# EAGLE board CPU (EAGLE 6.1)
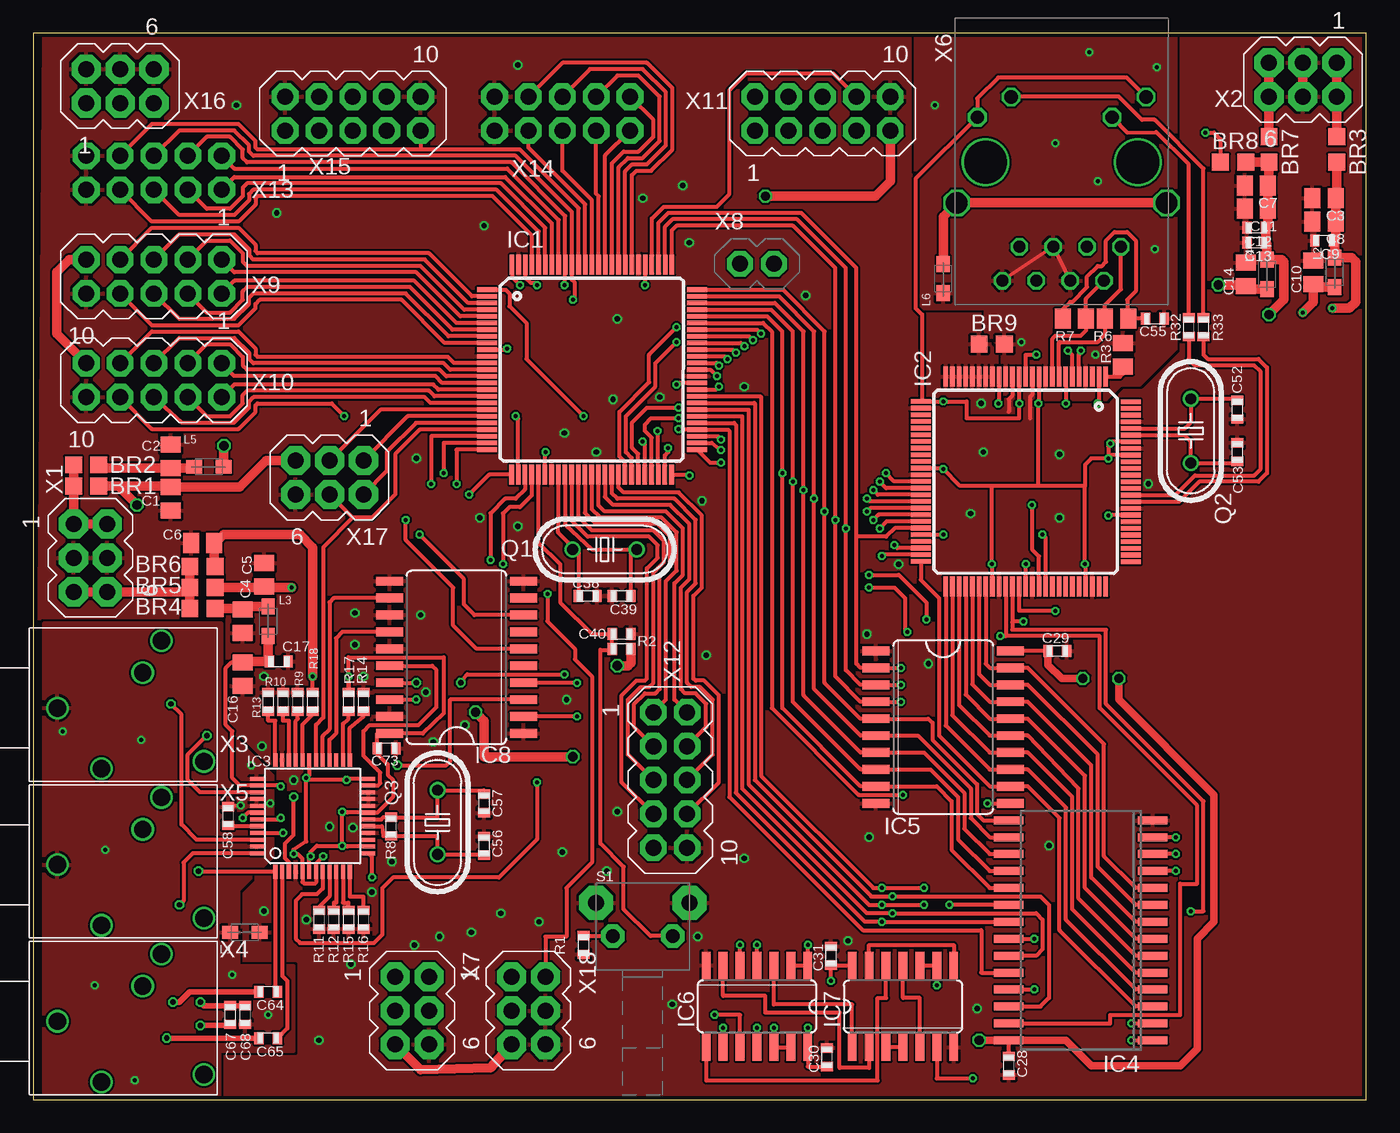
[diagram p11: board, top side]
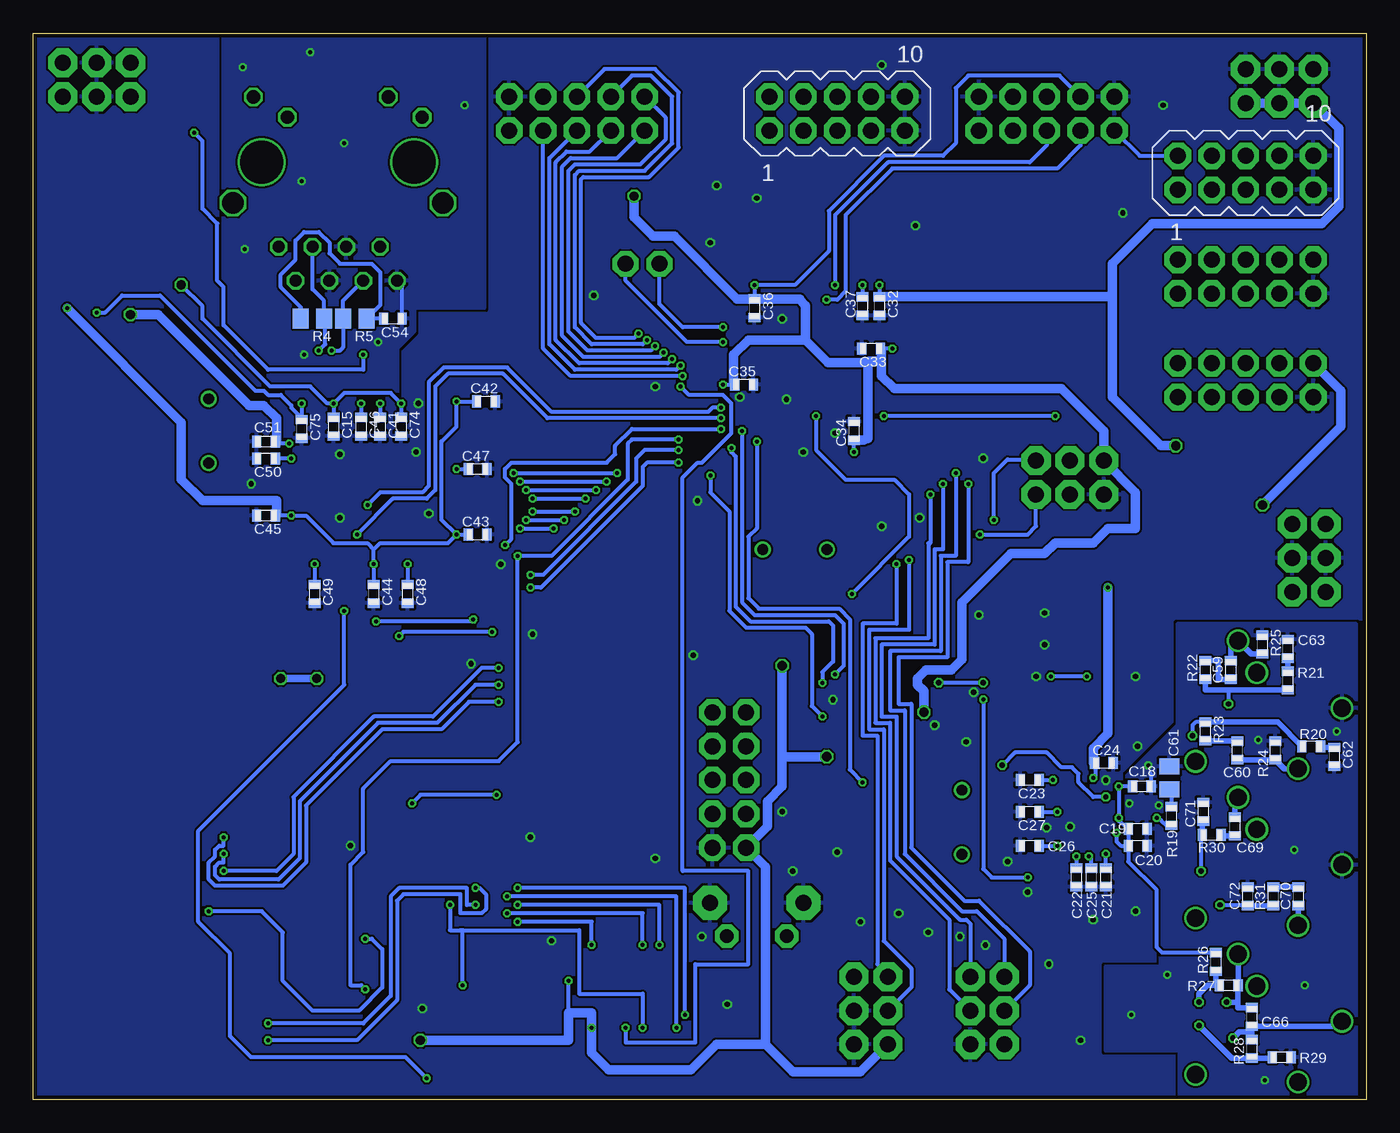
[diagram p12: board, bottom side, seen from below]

Size 100 x 80 mm. Coordinates in mm from the lower left corner, seen from the top.
Outline: 0,0 100,0 100,80 0,80 0,0
Copper layers (1*16): Top 0.035mm / dielectric 1.5mm / Bottom 0.035mm
Design rules: minimum track width 0.15mm, minimum drill 0.3mm, track to track 0.15mm, track to pad 0.15mm, pad to pad 0.15mm, via to via 0.15mm, smd to smd 0.15mm, copper to edge 0.3mm, drill to drill 0.2mm, minimum pad ring 0.2mm, minimum via ring 0.15mm, stop-mask expansion 0.075mm, vias tented up to drill 0mil, thermal gap 0.2mm

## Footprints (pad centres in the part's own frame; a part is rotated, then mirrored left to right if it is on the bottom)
0-OHM-BRÜCKE = smd 1.27 x 1.27: 1 -0.953,0; 2 0.953,0
0805 = smd 1.2 x 1.5: 1 -0.875,0; 2 0.875,0
0603 = smd 0.7 x 0.9: 1 -0.7,0; 2 0.7,0
TQFP100 = smd 1.5 x 0.35: 1 -7.875,6; 2 -7.875,5.5; 3 -7.875,5; 4 -7.875,4.5; 5 -7.875,4; 6 -7.875,3.5; 7 -7.875,3; 8 -7.875,2.5; 9 -7.875,2; 10 -7.875,1.5; 11 -7.875,1; 12 -7.875,0.5; 13 -7.875,0; 14 -7.875,-0.5; 15 -7.875,-1; 16 -7.875,-1.5; 17 -7.875,-2; 18 -7.875,-2.5; 19 -7.875,-3; 20 -7.875,-3.5; 21 -7.875,-4; 22 -7.875,-4.5; 23 -7.875,-5; 24 -7.875,-5.5; 25 -7.875,-6; 51 7.875,-6; 52 7.875,-5.5; 53 7.875,-5; 54 7.875,-4.5; 55 7.875,-4; 56 7.875,-3.5; 57 7.875,-3; 58 7.875,-2.5; 59 7.875,-2; 60 7.875,-1.5; 61 7.875,-1; 62 7.875,-0.5; 63 7.875,0; 64 7.875,0.5; 65 7.875,1; 66 7.875,1.5; 67 7.875,2; 68 7.875,2.5; 69 7.875,3; 70 7.875,3.5; 71 7.875,4; 72 7.875,4.5; 73 7.875,5; 74 7.875,5.5; 75 7.875,6 | smd 0.35 x 1.5: 26 -6.025,-7.875; 27 -5.525,-7.875; 28 -5.025,-7.875; 29 -4.525,-7.875; 30 -4.025,-7.875; 31 -3.525,-7.875; 32 -3.025,-7.875; 33 -2.525,-7.875; 34 -2.025,-7.875; 35 -1.525,-7.875; 36 -1.025,-7.875; 37 -0.525,-7.875; 38 -0.025,-7.875; 39 0.475,-7.875; 40 0.975,-7.875; 41 1.475,-7.875; 42 1.975,-7.875; 43 2.475,-7.875; 44 2.975,-7.875; 45 3.475,-7.875; 46 3.975,-7.875; 47 4.475,-7.875; 48 4.975,-7.875; 49 5.475,-7.875; 50 5.975,-7.875; 76 6,7.875; 77 5.5,7.875; 78 5,7.875; 79 4.5,7.875; 80 4,7.875; 81 3.5,7.875; 82 3,7.875; 83 2.5,7.875; 84 2,7.875; 85 1.5,7.875; 86 1,7.875; 87 0.5,7.875; 88 0,7.875; 89 -0.5,7.875; 90 -1,7.875; 91 -1.5,7.875; 92 -2,7.875; 93 -2.5,7.875; 94 -3,7.875; 95 -3.5,7.875; 96 -4,7.875; 97 -4.5,7.875; 98 -5,7.875; 99 -5.5,7.875; 100 -6,7.875
TQFP48 = smd 1.016 x 0.305: 1 -4.191,2.794; 2 -4.191,2.286; 3 -4.191,1.778; 4 -4.191,1.27; 5 -4.191,0.762; 6 -4.191,0.254; 7 -4.191,-0.254; 8 -4.191,-0.762; 9 -4.191,-1.27; 10 -4.191,-1.778; 11 -4.191,-2.286; 12 -4.191,-2.794; 25 4.191,-2.794; 26 4.191,-2.286; 27 4.191,-1.778; 28 4.191,-1.27; 29 4.191,-0.762; 30 4.191,-0.254; 31 4.191,0.254; 32 4.191,0.762; 33 4.191,1.27; 34 4.191,1.778; 35 4.191,2.286; 36 4.191,2.794 | smd 0.305 x 1.016: 13 -2.794,-4.191; 14 -2.286,-4.191; 15 -1.778,-4.191; 16 -1.27,-4.191; 17 -0.762,-4.191; 18 -0.254,-4.191; 19 0.254,-4.191; 20 0.762,-4.191; 21 1.27,-4.191; 22 1.778,-4.191; 23 2.286,-4.191; 24 2.794,-4.191; 37 2.794,4.191; 38 2.286,4.191; 39 1.778,4.191; 40 1.27,4.191; 41 0.762,4.191; 42 0.254,4.191; 43 -0.254,4.191; 44 -0.762,4.191; 45 -1.27,4.191; 46 -1.778,4.191; 47 -2.286,4.191; 48 -2.794,4.191
SOP28X = smd 0.6 x 2.2: 1 -8.255,-5.4; 2 -6.985,-5.4; 3 -5.715,-5.4; 4 -4.445,-5.4; 5 -3.175,-5.4; 6 -1.905,-5.4; 7 -0.635,-5.4; 8 0.635,-5.4; 9 1.905,-5.4; 10 3.175,-5.4; 11 4.445,-5.4; 12 5.715,-5.4; 13 6.985,-5.4; 14 8.255,-5.4; 15 8.255,5.4; 16 6.985,5.4; 17 5.715,5.4; 18 4.445,5.4; 19 3.175,5.4; 20 1.905,5.4; 21 0.635,5.4; 22 -0.635,5.4; 23 -1.905,5.4; 24 -3.175,5.4; 25 -4.445,5.4; 26 -5.715,5.4; 27 -6.985,5.4; 28 -8.255,5.4
SO20W = smd 0.66 x 2.032: 1 -5.715,-5.029; 2 -4.445,-5.029; 3 -3.175,-5.029; 4 -1.905,-5.029; 5 -0.635,-5.029; 6 0.635,-5.029; 7 1.905,-5.029; 8 3.175,-5.029; 9 4.445,-5.029; 10 5.715,-5.029; 11 5.715,5.029; 12 4.445,5.029; 13 3.175,5.029; 14 1.905,5.029; 15 0.635,5.029; 16 -0.635,5.029; 17 -1.905,5.029; 18 -3.175,5.029; 19 -4.445,5.029; 20 -5.715,5.029
SO14 = smd 0.66 x 2.032: 1 -3.81,-3.073; 2 -2.54,-3.073; 3 -1.27,-3.073; 4 0,-3.073; 5 1.27,-3.073; 6 2.54,-3.073; 7 3.81,-3.073; 8 3.81,3.073; 9 2.54,3.073; 10 1.27,3.073; 11 0,3.073; 12 -1.27,3.073; 13 -2.54,3.073; 14 -3.81,3.073
0805' = smd 1.2 x 1: 1 -1.1,0; 2 1.1,0
HC49U-V = drill 0.813: 1 -2.413,0; 2 2.413,0
PHAP3305 = drill 1 pad 1.778 octagon: 1 -2.25,-2.5; 2 2.25,-2.5 | drill 1.2 pad 2.54 octagon: SHD@0 -3.5,0; SHD@1 3.5,0
STIFTLEISTE-2X3PIN = drill 1.2 pad 2.184 octagon: 1 -2.54,-2.54; 2 0,-2.54; 3 2.54,-2.54; 4 -2.54,0; 5 0,0; 6 2.54,0
EBS35 = drill 1.3: GND -12,0; LEFT -4.2,5.05; LEFTGND -5.6,2.65; RIGHT -8.7,-4.55; RIGHTGND -1,-4
TRJ0011 = drill 0.9 octagon: 1 4.445,-6.35; 2 3.175,-8.89; 3 1.905,-6.35; 4 0.635,-8.89; 5 -0.635,-6.35; 6 -1.905,-8.89; 7 -3.175,-6.35; 8 -4.445,-8.89 | drill 1 octagon: 9 6.325,4.9; 10 3.785,3.38; 11 -3.785,4.9; 12 -6.325,3.38 | drill 3.2 pad 3.2: P$1 -5.715,0; P$2 5.715,0 | drill 1.6 octagon: SHD@0 -7.875,-3.05; SHD@1 7.875,-3.05
STIFTLEISTE-2PIN = drill 1.2 pad 1.93 octagon: 1 0,0; 2 2.54,0
STIFTLEISTE-2X5PIN = drill 1.2 pad 2 octagon: 1 -5.08,-2.54; 2 -2.54,-2.54; 3 0,-2.54; 4 2.54,-2.54; 5 5.08,-2.54; 6 -5.08,0; 7 -2.54,0; 8 0,0; 9 2.54,0; 10 5.08,0

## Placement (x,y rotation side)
BR1  0-OHM-BRÜCKE  [0-OHM-BRÜCKE]  3.97,46.04 0 top
BR2  0-OHM-BRÜCKE  [0-OHM-BRÜCKE]  3.97,47.62 0 top
BR3  0-OHM-BRÜCKE  [0-OHM-BRÜCKE]  97.79,71.28 270 top
BR4  0-OHM-BRÜCKE  [0-OHM-BRÜCKE]  12.7,36.83 0 top
BR5  0-OHM-BRÜCKE  [0-OHM-BRÜCKE]  12.7,38.42 0 top
BR6  0-OHM-BRÜCKE  [0-OHM-BRÜCKE]  12.7,40.01 0 top
BR7  0-OHM-BRÜCKE  [0-OHM-BRÜCKE]  92.71,71.28 270 top
BR8  0-OHM-BRÜCKE  [0-OHM-BRÜCKE]  90.01,70.33 0 top
BR9  0-OHM-BRÜCKE  [0-OHM-BRÜCKE]  71.91,56.67 0 top
C1  10µF  [0805]  10.32,45.09 270 top
C2  10µF  [0805]  10.32,48.26 90 top
C3  10µF  [0805]  96.84,67.63 180 top
C4  10µF  [0805]  15.72,35.88 270 top
C5  10µF  [0805]  17.3,39.37 90 top
C6  10µF  [0805]  12.7,41.75 180 top
C7  10µF  [0805]  91.76,68.58 180 top
C8  10µF  [0805]  96.84,65.88 180 top
C9  0µ1F  [0603]  96.84,64.45 180 top
C10  10µF  [0805]  96.04,62.07 90 top
C11  10µF  [0805]  91.76,66.83 180 top
C12  3µ3F  [0603]  91.76,65.41 180 top
C13  0µ1F  [0603]  91.76,64.29 180 top
C14  10µF  [0805]  90.96,61.91 90 top
C15  0µ1F  [0603]  77.47,50.48 270 bottom
C16  10µF  [0805]  15.72,31.91 270 top
C17  0µ1F  [0603]  18.41,32.86 0 top
C18  0µ1F  [0603]  16.83,23.5 0 bottom
C19  0µ1F  [0603]  17.14,20.32 0 bottom
C20  0µ1F  [0603]  17.14,19.05 0 bottom
C21  0µ1F  [0603]  19.53,16.67 270 bottom
C22  0µ1F  [0603]  21.75,16.67 270 bottom
C23  0µ1F  [0603]  25.24,23.97 180 bottom
C24  0µ1F  [0603]  19.68,25.24 0 bottom
C25  0µ1F  [0603]  20.64,16.67 270 bottom
C26  0µ1F  [0603]  25.24,19.05 180 bottom
C27  0µ1F  [0603]  25.24,21.59 180 bottom
C28  0µ1F  [0603]  73.18,2.54 270 top
C29  0µ1F  [0603]  76.83,33.66 0 top
C30  0µ1F  [0603]  59.53,3.17 90 top
C31  0µ1F  [0603]  59.85,10.79 90 top
C32  0µ1F  [0603]  36.51,59.53 270 bottom
C33  0µ1F  [0603]  37.15,56.36 180 bottom
C34  0µ1F  [0603]  38.42,50.16 90 bottom
C35  0µ1F  [0603]  46.67,53.66 0 bottom
C36  0µ1F  [0603]  45.88,59.37 270 bottom
C37  0µ1F  [0603]  37.78,59.53 270 bottom
C38  22pF  [0603]  41.59,37.78 0 top
C39  22pF  [0603]  44.13,37.78 180 top
C40  0µ1F  [0603]  44.13,34.92 0 top
C41  0µ1F  [0603]  73.98,50.48 270 bottom
C42  0µ1F  [0603]  66.04,52.39 0 bottom
C43  0µ1F  [0603]  66.67,42.39 0 bottom
C44  0µ1F  [0603]  74.45,37.94 270 bottom
C45  0µ1F  [0603]  82.55,43.81 180 bottom
C46  0µ1F  [0603]  75.41,50.48 270 bottom
C47  0µ1F  [0603]  66.67,47.31 0 bottom
C48  0µ1F  [0603]  71.91,37.94 270 bottom
C49  0µ1F  [0603]  78.9,37.94 270 bottom
C50  0µ1F  [0603]  82.55,48.1 180 bottom
C51  0µ1F  [0603]  82.55,49.37 180 bottom
C52  22pF  [0603]  90.33,51.75 90 top
C53  22pF  [0603]  90.33,48.58 270 top
C54  0µ1F  [0603]  73.03,58.58 180 bottom
C55  0µ1F  [0603]  84.14,58.58 0 top
C56  33pF  [0603]  33.81,19.05 90 top
C57  33pF  [0603]  33.81,22.23 270 top
C58  1µF  [0603]  14.61,21.27 90 top
C59  1µF  [0603]  10.16,32.23 90 bottom
C60  1µF  [0603]  9.68,26.19 270 bottom
C61  47nF  [0805]  14.76,24.13 90 bottom
C62  10nF  [0603]  2.38,25.72 270 bottom
C63  10nF  [0603]  5.87,33.81 90 bottom
C64  1µF  [0603]  17.62,8.1 180 top
C65  1µF  [0603]  17.62,4.6 180 top
C66  100pF  [0603]  8.57,6.19 270 bottom
C67  10µF  [0603]  14.76,6.35 270 top
C68  10µF  [0603]  15.88,6.35 270 top
C69  1µF  [0603]  9.84,20.48 90 bottom
C70  1µF  [0603]  5.08,15.24 270 bottom
C71  10nF  [0603]  12.22,21.59 90 bottom
C72  10nF  [0603]  8.89,15.24 90 bottom
C73  0µ1F  [0603]  26.51,26.35 0 top
C74  0µ1F  [0603]  72.39,50.48 270 bottom
C75  0µ1F  [0603]  79.85,50.32 270 bottom
IC1  ATMEGA-2560  [TQFP100]  41.91,54.77 0 top
IC2  W5300  [TQFP100]  74.45,46.35 270 top
IC3  VS1053B  [TQFP48]  20.95,21.27 90 top
IC4  62256-70M  [SOP28X]  78.58,12.7 90 top
IC5  74VHC573D  [SO20W]  68.26,27.94 270 top
IC6  7400  [SO14]  54.29,6.99 180 top
IC7  7400  [SO14]  65.25,6.99 0 top
IC8  74HCT244DW  [SO20W]  31.75,33.18 90 top
L1  1µH  [0805']  15.88,12.54 0 top
L2  1µH  [0805']  97.63,62.07 270 top
L3  1µH  [0805']  17.62,35.88 270 top
L4  1µH  [0805']  92.55,61.91 270 top
L5  10µH  [0805']  13.18,47.47 0 top
L6  120R Ferrit  [0805']  68.26,61.59 90 top
Q1  16 MHz  [HC49U-V]  42.86,41.27 0 top
Q2  25MHz  [HC49U-V]  86.84,50.16 270 top
Q3  12.288  [HC49U-V]  30.32,20.8 90 top
R1  100R  [0603]  41.27,11.59 90 top
R2  10K  [0603]  44.13,33.81 180 top
R3  12K3  [0805]  81.76,55.88 90 top
R4  49R9  [0805]  79.06,58.58 180 bottom
R5  49R9  [0805]  75.88,58.58 0 bottom
R6  49R9  [0805]  81.28,58.58 180 top
R7  49R9  [0805]  78.11,58.58 0 top
R8  1M  [0603]  26.83,20.48 90 top
R9  100K  [0603]  19.84,29.84 270 top
R10  100K  [0603]  18.73,29.84 270 top
R11  100K  [0603]  21.43,13.49 90 top
R12  100K  [0603]  22.54,13.49 90 top
R13  100K  [0603]  17.62,29.84 270 top
R14  100K  [0603]  24.77,29.84 270 top
R15  100K  [0603]  23.65,13.49 90 top
R16  100K  [0603]  24.77,13.49 90 top
R17  100K  [0603]  23.65,29.84 270 top
R18  100K  [0603]  20.95,29.84 270 top
R19  10R  [0603]  14.61,21.27 270 bottom
R20  22R  [0603]  4.13,26.51 180 bottom
R21  22R  [0603]  5.87,31.43 270 bottom
R22  100R  [0603]  12.06,32.23 90 bottom
R23  100R  [0603]  12.06,27.62 270 bottom
R24  10K  [0603]  6.83,26.19 270 bottom
R25  10K  [0603]  7.78,34.13 270 bottom
R26  1K  [0603]  11.27,10.32 90 bottom
R27  1K  [0603]  10.32,8.57 180 bottom
R28  1K  [0603]  8.57,3.81 90 bottom
R29  1K  [0603]  6.35,3.17 180 bottom
R30  470R  [0603]  11.59,19.84 0 bottom
R31  470R  [0603]  6.99,15.24 90 bottom
R32  220R  [0603]  86.68,57.94 90 top
R33  220R  [0603]  87.79,57.94 90 top
S1  PHAP3305  [PHAP3305]  45.72,14.76 0 top
X1  VIN  [STIFTLEISTE-2X3PIN]  5.56,40.64 270 top
X2  VIN  [STIFTLEISTE-2X3PIN]  95.25,75.25 180 top
X3  DS_1503_09  [EBS35]  13.81,29.37 0 top
X4  DS_1503_09  [EBS35]  13.81,5.87 0 top
X5  DS_1503_09  [EBS35]  13.81,17.62 0 top
X6  TRJ0011  [TRJ0011]  77.15,70.33 0 top
X7  PB  [STIFTLEISTE-2X3PIN]  29.69,6.67 270 top
X8  TWI  [STIFTLEISTE-2PIN]  53.02,62.71 0 top
X9  PE  [STIFTLEISTE-2X5PIN]  9.05,60.48 180 top
X10  PH  [STIFTLEISTE-2X5PIN]  9.05,52.7 180 top
X11  PJ  [STIFTLEISTE-2X5PIN]  59.21,75.25 0 top
X12  PL  [STIFTLEISTE-2X5PIN]  49.05,23.97 270 top
X13  PF  [STIFTLEISTE-2X5PIN]  9.05,70.8 0 bottom
X14  PK  [STIFTLEISTE-2X5PIN]  39.69,75.25 0 bottom
X15  JTAG  [STIFTLEISTE-2X5PIN]  23.97,75.25 0 top
X16  ADC Supply  [STIFTLEISTE-2X3PIN]  6.51,77.31 0 top
X17  SPI  [STIFTLEISTE-2X3PIN]  22.23,45.4 180 top
X18  PG  [STIFTLEISTE-2X3PIN]  38.42,6.67 270 top

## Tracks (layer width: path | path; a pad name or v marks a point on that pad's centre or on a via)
1V8O  (via drill 0.3)
  Top 0.3: IC2.13 74.45,55.88 v75.25,55.88 | v87.95,72.55 88.58,72.55 89.06,72.07 BR8.1
  Bottom 0.3: v75.25,55.88 75.25,54.77 82.39,54.77 85.72,58.1 85.72,60.96 86.2,61.44 86.2,65.72 87.31,66.83 87.31,71.91 v87.95,72.55
3V3
  Top 0.7: X2.1 X2.4 BR3.1
!FDX
  Top 0.3: IC2.86 85.68,45.35 87.15,46.83 91.6,46.83 92.08,47.31 92.08,54.61 91.6,55.09 87.15,55.09 86.68,55.56 R32.1
!RD  (via drill 0.3)
  Top 0.3: IC1.52 50.9,49.27 v51.59,48.74 | IC4.22 v75.09,12.06 | v86.84,14.13 87.79,14.13 87.79,22.38 80.49,29.69 80.49,35.24 73.45,35.24 73.45,35.83 | IC2.61 73.45,35.83 | v62.71,39.37 64.93,39.37 66.99,37.31 v66.99,36.04 | v74.3,35.88 73.5,35.88 73.45,35.83
  Bottom 0.3: v51.59,48.74 54.13,48.74 54.77,48.1 54.77,46.35 61.75,39.37 v62.71,39.37 | v75.09,12.06 74.61,12.06 73.82,11.27 73.82,8.41 75.56,6.67 79.06,6.67 81.28,8.89 81.28,12.54 82.87,14.13 v86.84,14.13 | v66.99,36.04 67.15,35.88 v74.3,35.88
!SPD
  Top 0.3: R33.1 87.79,55.88 88.11,55.56 91.92,55.56 92.55,54.93 92.55,46.99 91.92,46.35 87.47,46.35 85.97,44.85 IC2.85
!WR  (via drill 0.3)
  Top 0.3: IC4.27 80.8,5.71 80.8,6.35 86.04,6.35 86.04,16.19 87.31,16.19 87.31,22.07 80.01,29.37 80.01,34.77 72.95,34.77 | IC2.60 72.95,34.77 | IC1.51 50.77,47.78 v51.59,47.78 | v62.71,38.42 64.61,38.42 65.41,37.62 65.41,35.24 v65.56,35.08 | v72.55,34.77 72.95,34.77
  Bottom 0.3: v51.59,47.78 53.98,47.78 54.29,47.47 54.29,46.04 61.91,38.42 v62.71,38.42 | v65.56,35.08 72.23,35.08 v72.55,34.77
+1V8
  Top 0.7: X2.3 X2.6 BR7.1
+3V3
  Top 0.7: X1.3 X1.6 11.43,38.1 BR5.1 | BR5.1 BR4.1 | BR5.1 BR6.1
+5V
  Top 0.7: BR2.1 BR1.1 X1.1 X1.4
A0
  Top 0.3: IC2.57 71.45,32.69 71.75,32.38 IC5.19 74.61,32.38 80.33,26.67 80.33,18.26 82.71,15.88 IC4.10
A1
  Top 0.3: IC2.56 70.95,31.92 71.75,31.11 IC5.18 74.61,31.11 79.85,25.88 79.85,17.46 82.71,14.61 IC4.9
A2
  Top 0.3: IC2.55 70.45,31.15 71.75,29.84 IC5.17 74.61,29.84 79.38,25.08 79.38,16.67 82.71,13.34 IC4.8
A3
  Top 0.3: IC2.54 69.95,30.38 71.75,28.57 IC5.16 74.61,28.57 78.9,24.29 78.9,15.88 82.71,12.06 IC4.7
A4
  Top 0.3: IC2.53 69.45,29.61 71.75,27.3 IC5.15 74.61,27.3 78.42,23.34 78.42,15.08 82.71,10.79 IC4.6
A5
  Top 0.3: IC2.52 68.95,28.84 71.75,26.04 IC5.14 74.61,26.04 77.95,22.7 77.95,14.29 82.71,9.53 IC4.5
A6
  Top 0.3: IC2.51 68.45,28.07 71.75,24.77 IC5.13 74.61,24.77 77.47,21.91 77.47,13.49 82.71,8.26 IC4.4
A7
  Top 0.3: IC2.50 66.58,38.99 67.94,37.62 67.94,27.3 71.75,23.5 IC5.12 74.61,23.5 76.99,21.11 76.99,12.7 82.71,6.99 IC4.3
A8  (via drill 0.3)
  Top 0.3: IC2.49 63.74,40.88 v63.66,40.8 | IC1.53 51.35,49.77 v51.59,49.53 | IC4.25 v75.09,8.26
  Bottom 0.3: v51.59,49.53 55.09,49.53 55.4,49.21 55.4,46.51 61.12,40.8 v63.66,40.8 63.66,26.83 65.09,25.4 73.18,25.4 75.25,23.34 75.25,18.57 76.2,17.62 76.2,8.57 75.41,8.57 v75.09,8.26
A9  (via drill 0.3)
  Top 0.3: IC4.24 71.12,9.53 71.12,12.7 62.23,12.7 52.23,22.7 52.23,50.16 52.12,50.27 IC1.54 48.47,50.27 v48.42,50.32 | IC2.48 64.82,41.38 v64.61,41.59
  Bottom 0.3: v64.61,41.59 64.14,42.07 64.14,46.2 64.61,46.67 64.61,47.31 64.14,47.78 56.99,47.78 56.36,48.42 56.36,49.05 55.09,50.32 v48.42,50.32
A10  (via drill 0.3)
  Top 0.3: IC1.55 52.58,50.77 52.7,50.64 52.7,23.02 62.39,13.34 v63.66,13.34 IC4.21 | IC6.2 IC6.1 v58.1,11.59
  Bottom 0.3: v58.1,11.59 58.1,13.34 v63.66,13.34
A11  (via drill 0.3)
  Top 0.3: IC1.56 53.17,51.27 53.18,51.28 53.18,23.34 62.55,13.97 v64.45,13.97 75.25,13.97 75.72,13.49 75.72,11.27 75.25,10.79 IC4.23 | IC6.4 v54.29,11.59
  Bottom 0.3: v54.29,11.59 54.29,13.97 v64.45,13.97
A12  (via drill 0.3)
  Top 0.3: IC1.57 53.64,51.77 53.66,51.75 53.66,23.65 62.71,14.61 v63.66,14.61 v66.83,14.61 | v82.39,5.71 IC4.2 | IC6.5 v53.02,11.59
  Bottom 0.3: v66.83,14.61 67.47,14.61 67.47,15.88 72.55,15.88 73.18,15.24 73.18,7.78 75.25,5.71 v82.39,5.71 | v53.02,11.59 53.02,14.61 v63.66,14.61
A13  (via drill 0.3)
  Top 0.3: IC1.58 54.09,52.27 54.13,52.23 54.13,23.97 62.87,15.24 v64.45,15.24 75.56,15.24 76.2,14.61 76.2,7.62 75.56,6.99 IC4.26 | IC6.9 v51.75,5.4
  Bottom 0.3: v51.75,5.4 51.75,15.24 v64.45,15.24
A14  (via drill 0.3)
  Top 0.3: IC1.59 54.55,52.77 54.61,52.7 54.61,24.29 63.02,15.88 v63.66,15.88 v66.83,15.88 | v82.39,4.45 IC4.1 | IC6.10 53.02,6.35 v51.12,6.35
  Bottom 0.3: v66.83,15.88 66.52,15.88 66.04,15.4 66.04,14.29 66.36,13.97 67.94,13.97 67.94,15.4 72.23,15.4 72.71,14.92 72.71,7.46 75.72,4.45 v82.39,4.45 | v51.12,6.35 51.12,15.88 v63.66,15.88
A15  (via drill 0.3)
  Top 0.3: IC6.13 IC6.12 v55.56,5.4 | 51.28,53.34 v51.44,53.5 51.2,53.27 IC1.60
  Bottom 0.3: v55.56,5.4 55.56,4.29 50.32,4.29 50.32,10.16 46.35,10.16 46.35,17.14 51.28,17.14 51.28,46.67 50.16,47.78 49.85,47.78 47.62,50.01 47.62,52.23 48.26,52.86 50.8,52.86 v51.44,53.5
AD0  (via drill 0.3)
  Top 0.3: 61.75,42.23 61.75,32.7 62.07,32.38 IC5.2 v65.09,32.38 | 61.75,42.23 61.75,62.39 57.63,66.52 47.62,66.52 46.91,65.8 IC1.78 | IC2.45 64.63,42.88 63.98,42.23 61.75,42.23 | v85.72,17.14 IC4.11
  Bottom 0.3: v65.09,32.38 66.36,32.38 70.01,28.73 74.45,28.73 80.49,22.7 80.49,18.41 81.76,17.14 v85.72,17.14
AD1  (via drill 0.3)
  Top 0.3: IC1.77 47.41,65.51 47.94,66.04 57.31,66.04 60.96,62.39 v60.96,42.86 60.96,32.23 62.07,31.11 IC5.3 v65.09,31.11 | IC2.44 64.02,43.38 v63.5,42.86 | v85.72,18.41 IC4.12
  Bottom 0.3: v63.5,42.86 v60.96,42.86 | v65.09,31.11 66.83,31.11 69.69,28.26 74.14,28.26 80.01,22.38 80.01,18.1 81.6,16.51 86.04,16.51 86.36,16.83 86.36,17.46 86.04,17.78 85.72,17.78 v85.72,18.41
AD2  (via drill 0.3)
  Top 0.3: IC1.76 47.91,65.21 48.26,65.56 56.99,65.56 60.17,62.39 v60.17,43.5 60.17,31.75 62.07,29.84 IC5.4 v65.09,29.84 | IC2.43 63.41,43.88 v63.02,43.5 | v85.72,19.68 IC4.13
  Bottom 0.3: v63.02,43.5 v60.17,43.5 | v65.09,29.84 67.31,29.84 69.37,27.78 73.82,27.78 79.53,22.07 79.53,17.78 81.28,16.03 86.36,16.03 86.84,16.51 86.84,17.78 86.36,18.26 86.36,18.73 86.04,19.05 85.72,19.05 v85.72,19.68
AD3  (via drill 0.3)
  Top 0.3: IC1.75 56.23,60.77 59.37,57.63 v59.37,44.13 59.37,31.27 62.07,28.57 IC5.5 67.15,28.57 67.47,28.26 67.47,26.99 70.8,23.65 70.8,21.43 71.28,20.95 IC4.15 | IC2.42 62.8,44.38 v62.55,44.13
  Bottom 0.3: v62.55,44.13 v59.37,44.13
AD4  (via drill 0.3)
  Top 0.3: IC1.74 55.94,60.27 58.58,57.63 v58.58,45.09 58.58,30.8 62.07,27.3 IC5.6 66.36,27.3 70.33,23.34 70.33,21.11 71.75,19.68 IC4.16 | IC2.41 62.75,44.88 v62.55,45.09
  Bottom 0.3: v62.55,45.09 v58.58,45.09
AD5  (via drill 0.3)
  Top 0.3: IC1.73 55.64,59.77 57.78,57.63 v57.78,45.72 57.78,30.32 62.07,26.04 IC5.7 66.83,26.04 69.85,23.02 69.85,20.32 71.75,18.41 IC4.17 | IC2.40 63.36,45.38 v63.02,45.72
  Bottom 0.3: v63.02,45.72 v57.78,45.72
AD6  (via drill 0.3)
  Top 0.3: IC1.72 55.35,59.27 56.99,57.63 v56.99,46.35 56.99,29.84 62,24.84 arc45 62.18,24.77 IC5.8 67.31,24.77 69.37,22.7 69.37,19.53 71.75,17.14 IC4.18 | IC2.39 63.98,45.88 v63.5,46.35
  Bottom 0.3: v63.5,46.35 v56.99,46.35
AD7  (via drill 0.3)
  Top 0.3: IC1.71 55.05,58.77 56.2,57.63 v56.2,46.99 56.2,29.37 62.07,23.5 IC5.9 67.79,23.5 68.9,22.38 68.9,18.73 71.75,15.88 IC4.19 | IC2.38 64.59,46.38 v63.98,46.99
  Bottom 0.3: v63.98,46.99 v56.2,46.99
ADC0
  Top 0.3: IC1.97 37.41,64.83 34.45,67.79 16.83,67.79 16.67,67.63 16.67,67.15 15.4,65.88 8.89,65.88 X13.4
ADC1
  Top 0.3: IC1.96 37.91,65.12 34.77,68.26 16.51,68.26 16.19,67.94 16.19,67.47 15.08,66.36 10.95,66.36 X13.3
ADC2
  Top 0.3: IC1.95 38.41,65.41 35.08,68.74 16.03,68.74 15.72,68.42 15.72,67.79 14.76,66.83 13.02,66.83 X13.2
ADC3
  Top 0.3: X13.1 15.08,69.22 35.4,69.22 38.91,65.71 IC1.94
ADC4
  Top 0.3: X13.6 15.08,69.85 35.56,69.85 39.41,66 IC1.93
  Bottom 0.3: X15.1 16.99,70.8 X13.6
ADC5  (via drill 0.3)
  Top 0.3: X13.7 13.02,72.23 14.76,72.23 15.72,71.28 15.72,70.64 16.03,70.33 35.88,70.33 39.91,66.29 IC1.92 39.91,61.18 v39.85,61.12
  Bottom 0.3: X15.3 23.97,71.6 25.24,70.33 35.88,70.33 39.85,66.36 v39.85,61.12
ADC6  (via drill 0.3)
  Top 0.3: X13.8 10.95,72.71 15.08,72.71 16.19,71.6 16.19,71.12 16.51,70.8 36.2,70.8 40.41,66.59 IC1.91 40.41,61.51 40.64,61.28 40.64,60.17 v40.48,60.01
  Bottom 0.3: X15.2 21.43,71.6 23.18,69.85 35.56,69.85 39.05,66.36 39.05,60.64 39.69,60.01 v40.48,60.01
ADC7
  Top 0.3: IC1.90 40.91,66.88 36.51,71.28 29.05,71.28 | 29.05,71.28 16.83,71.28 16.67,71.44 16.67,71.91 15.4,73.18 8.89,73.18 X13.9 | X15.5 29.05,71.28
ADC8
  Top 0.3: IC1.89 41.41,67.17 37.15,71.44 X14.4
ADC9
  Top 0.3: IC1.88 41.91,67.47 39.69,69.69 X14.3
ADC10
  Top 0.3: IC1.87 42.41,67.76 42.23,67.94 X14.2
ADC11
  Top 0.3: IC1.86 42.91,70.85 X14.1
ADC12
  Top 0.3: IC1.85 43.41,70.24 44.29,71.12 45.4,71.12 46.51,72.23 46.51,73.5 X14.6
ADC13
  Top 0.3: IC1.84 43.91,69.94 44.61,70.64 45.72,70.64 46.99,71.91 46.99,75.25 45.4,76.83 43.81,76.83 X14.7
ADC14
  Top 0.3: IC1.83 44.41,69.65 44.93,70.17 46.04,70.17 47.47,71.6 47.47,75.56 45.72,77.31 41.75,77.31 X14.8
ADC15
  Top 0.3: IC1.82 44.91,69.36 45.24,69.69 46.35,69.69 47.94,71.28 47.94,75.88 46.04,77.79 39.69,77.79 X14.9
AGND  (via drill 0.3)
  Top 0.3: C58.2 14.86,22.07 v15.56,22.07
  Bottom 0.3: C18.2 16.13,24.38 16.19,24.45
  other vias: 14.92,9.37 17.62,6.35 7.62,1.43 4.6,8.57 5.4,18.73 8.1,26.99 2.22,27.62 17.78,22.23 16.35,25.08
  pour Bottom: 0.79,0.16 13.97,0.16 13.97,3.65 19.53,3.65 19.53,10 15.4,10 15.4,15.72 17.94,18.26 17.94,24.29 14.13,28.1 14.13,35.72 0.79,35.72
  pour Top: 0.79,0.16 13.97,0.16 13.97,3.65 19.53,3.65 19.53,10 15.4,10 15.4,15.72 17.94,18.26 17.94,24.29 14.13,28.1 14.13,35.72 0.79,35.72
ALE  (via drill 0.3)
  Top 0.3: IC1.70 54.76,58.27 55.4,57.63 55.4,29.37 61.91,22.86 v65.25,22.86 | v71.6,22.23 IC5.11
  Bottom 0.3: v65.25,22.86 70.96,22.86 v71.6,22.23
AVCC  (via drill 0.3, 0.7)
  Top 0.3: IC1.100 35.91,61.72 v36.51,61.12
  Top 0.7: L5.2 14.28,49.04 v14.29,49.05
  Bottom 0.3: v36.51,61.12 C32.1
  Bottom 0.7: v14.29,49.05 15.4,49.05 19.05,52.7 19.05,60.23 | X16.3 X16.2 X16.1 2.06,72.87 2.06,66.99 3.33,65.72 16.03,65.72 19.05,62.71 19.05,60.23 | 19.05,60.23 C32.1
AVDD  (via drill 0.3)
  Top 0.3: v18.57,23.5 18.35,23.56 IC3.38 15.49,23.56 14.92,24.13 14.92,27.62 14.45,28.1 14.45,32.38 14.85,32.78 C16.1 | IC3.43 18.35,21.02 v18.57,21.11 | IC3.45 v18.73,20
  Top 0.7: L3.2 17.62,32.95 C17.1 15.79,32.86 C16.1
  Bottom 0.3: C18.1 v18.57,23.5 v18.57,21.11 18.57,20.89 C19.1 C20.1 | v18.73,20 18.73,19.37 18.41,19.05 C20.1 | R26.2 15.3,11.02 15.72,11.43 15.72,15.72 17.84,17.84 C20.1
CVDD  (via drill 0.3)
  Top 0.3: IC3.31 20.7,24.35 v20.48,24.13 | IC3.24 23.59,24.07 v23.5,23.97 20.48,23.97 v20.48,24.13 | v20.48,24.13 20.48,19.37 19.53,18.73 v19.53,18.41 19.84,18.41 20.19,18.07 IC3.5 20.19,16.32 20.32,16.19 21.11,16.19 21.21,16.29 IC3.7 21.21,17.72 v21.75,18.26
  Top 0.7: BR5.2 17.23,38.42 | 17.23,38.42 C5.1 | 17.23,38.42 v19.37,38.42
  Bottom 0.3: v20.48,24.13 20.32,24.29 20.32,25.18 C24.1 | C23.1 v23.5,23.97 | C21.1 v19.53,18.41 | v21.75,18.26 C22.1
  Bottom 0.7: v19.37,38.42 19.37,27.46 20.48,26.35 20.48,25.24 C24.1
DVDD  (via drill 0.3)
  Top 0.3: IC3.6 20.7,18.16 v20.8,18.26 20.8,18.57 21.27,19.05 v23.18,19.05 | IC3.14 23.56,18.99 v23.18,19.05 | v23.18,19.05 v23.18,21.59 23.56,21.53 IC3.19 25.81,21.53 26.99,22.7 26.99,23.97 26.59,24.37 26.59,25.16 25.81,25.94 C73.1 25.81,27.46 IC8.20 29.21,27.46 30.8,28.97 30.8,33.18 23.65,33.18 R17.1 v23.65,31.75 | R18.1 v20.95,31.75
  Top 0.55: 13.65,41.75 C6.1
  Top 0.7: C6.1 13.57,40.08 BR6.2 | v20.95,31.75 20.95,41.43 20,42.39 14.29,42.39 13.65,41.75
  Bottom 0.3: C25.1 20.64,18.1 v20.8,18.26 | C27.1 v23.18,21.59 | C26.1 v23.18,19.05 | v20.95,31.75 v23.65,31.75
GND  (via drill 0.4)
  Top 0.3: IC2.12 74.95,52.89 74.77,52.7 74.77,51.12 | IC2.15 73.45,52.82 73.18,52.55 73.18,51.59
  Top 0.7: X2.2 X2.5
  other vias: 24.77,31.75 17.3,14.13 22.23,20.48 30,26.83 32.38,28.1 25.4,15.56 20.48,13.49 70.33,43.97 76.99,43.66 76.99,48.42 71.28,48.58 83.66,46.2 24.13,34.13 24.13,36.51 29.05,36.35 17.3,31.75 17.14,26.51 19.53,23.97 23.97,20.4 26.91,17.86 29.45,30.56 21.43,4.45 28.57,11.59 30.48,12.22 32.86,12.54 23.81,10.16 35.08,13.97 37.94,13.34 39.69,18.57 28.73,48.1 33.5,43.66 36.35,43.02 45.72,67.63 36.35,77.63 33.81,65.56 18.26,66.52 15.24,74.61 48.74,68.58 61.12,11.91 62.71,19.68 53.34,18.1 70.8,6.83 76.2,19.05 43.5,52.55 39.85,50.01 42.23,48.58 43.81,58.58 53.34,53.5 57.94,60.33 50.16,44.93 50.48,33.34 40.01,30 43.02,17.14 43.81,21.59 67.15,32.7 62.55,34.92 64.93,40.16 47.94,7.14 49.85,12.22 49.21,64.29 71.12,52.23 46.99,52.7
  pour Top (rank 2): 0.79,79.76 0.16,0.16 99.77,0.16 99.77,79.76
  pour Bottom (rank 2): 0.16,79.76 0.16,0.16 99.77,0.16 99.77,79.76
GNDA  (via drill 0.3)
  Top 0.3: X6.4 X6.5 X6.8
  Bottom 0.3: C54.1 72.33,61.05 X6.8
  other vias: 79.69,55.88 74.14,56.83 67.63,74.61 76.68,71.75 79.22,78.58 84.3,77.47 79.85,68.9 84.14,63.82
  pour Top: 72.71,52.55 80.49,52.55 81.6,53.66 83.03,53.66 85.72,56.36 85.72,80.01 66.2,80.01 66.2,59.37 71.44,59.37 71.44,57.63 72.71,56.36
  pour Bottom: 72.71,52.55 80.49,52.55 81.6,53.66 83.03,53.66 85.72,56.36 85.72,80.01 66.2,80.01 66.2,59.37 71.44,59.37 71.44,57.63 72.71,56.36
N$1
  Top 0.7: BR4.2 15.64,36.83 C4.1 15.94,36.98 L3.1
N$2
  Top 0.55: 12.06,47.47 L5.1
  Top 0.7: BR2.2 5.16,47.38 C2.1 11.98,47.38 12.06,47.47
N$3
  Top 0.3: IC1.34 39.88,43.14 41.91,41.27 Q1.2 44.83,40.99 C39.1
N$4
  Top 0.3: IC1.33 39.38,44.59 39.37,43.02 39.37,42.55 40.45,41.47 Q1.1 40.89,41.15 C38.1
N$5  (via drill 0.3)
  Top 0.3: IC1.98 36.91,61.67 37.31,61.28 37.62,61.28 v37.78,61.12
  Bottom 0.3: v37.78,61.12 C37.1
N$6
  Top 0.3: IC1.30 37.88,41.81 39.53,40.16 39.53,37.31 41.91,34.92 C40.1 | S1.2 46.31,12.26 44.29,14.29 44.29,17.46 42.55,19.21 42.55,33.75 43.37,33.75 R2.2 C40.1 | C40.1 43.5,34.92
N$7
  Top 0.3: R1.2 43.45,12.29 S1.1
N$8
  Top 0.3: IC7.1 61.44,7.14 55.56,7.14 IC6.3
N$9
  Top 0.3: IC7.2 62.71,2.38 60.48,2.38 60.48,6.51 54.93,6.51 54.93,7.78 51.75,7.78 IC6.6
N$10
  Top 0.3: IC7.4 IC7.3
N$11
  Top 0.3: IC6.8 50.48,1.43 63.34,1.43 63.34,7.62 63.98,7.62 IC7.12
N$12
  Top 0.3: IC7.13 62.71,11.59 69.06,11.59 IC7.8
N$13
  Top 0.3: IC7.5 66.52,7.62 65.25,7.62 IC7.11
N$14
  Top 0.3: IC2.95 86.35,49.85 86.84,49.37 Q2.2 90.2,47.75 C53.2
N$15
  Top 0.3: IC2.96 86.39,50.35 86.84,50.8 Q2.1 90.2,52.58 C52.2
N$16
  Top 0.3: IC2.1 81.53,54.23 81.76,54.45 R3.1
N$17
  Top 0.3: R7.1 77.23,59.29 77.79,59.85 77.95,59.85 79.06,60.96 79.06,61.75 79.85,62.55 80.17,62.55 80.49,62.87 80.49,64.45 81.12,65.09 82.07,65.09 82.71,64.45 82.71,60.64 82.07,60.01 82.07,58.66 R6.1 C55.1
N$18
  Bottom 0.3: R4.2 79.93,59.45 81.44,60.96 81.44,61.91 80.33,63.02 80.33,64.45 79.69,65.09 78.58,65.09 77.79,64.29 77.79,63.5 76.99,62.71 74.61,62.71 73.98,62.07 73.98,59.61 R5.2 C54.2
N$19
  Top 0.3: IC3.12 23.75,15.24 24.77,15.24 R16.2
N$20
  Top 0.3: IC3.11 23.24,14.76 23.65,14.76 R15.2
N$21
  Top 0.3: IC3.25 23.75,27.88 24.77,28.73 R14.2
N$22
  Top 0.3: IC3.36 18.16,28.42 17.62,28.42 R13.2
N$23
  Top 0.3: IC3.10 22.73,14.76 22.54,14.76 R12.2
N$24
  Top 0.3: IC3.9 22.23,15.24 21.43,14.45 R11.2
N$25
  Top 0.3: IC3.34 19.18,28.42 18.73,28.42 R10.2
N$26
  Top 0.3: IC3.33 19.68,28.42 19.84,28.57 R9.2
N$27
  Top 0.3: IC3.17 26.16,20.51 26.26,19.78 R8.1 30.32,19.78 Q3.1 33.81,18.38 C56.1
N$28
  Top 0.3: IC3.18 26.1,21.02 26.26,21.18 R8.2 30.32,21.18 Q3.2 33.81,23.21 C57.1
N$29
  Top 0.3: IC3.32 20.19,28.13 20.95,28.89 R18.2
N$30
  Top 0.3: IC3.26 23.24,28.19 23.65,28.57 R17.2
N$31
  Top 0.3: IC3.44 14.67,20.51 C58.1
N$32  (via drill 0.4)
  Top 0.3: IC3.46 12.26,19.49 11.11,20.64 11.11,28.89 v10.32,29.69
  Bottom 0.3: v10.32,29.69 10.32,30.73
  Bottom 0.406: R21.2 10.32,30.73 12.06,30.73 R22.1
N$33  (via drill 0.4)
  Top 0.3: IC3.39 12.51,23.05 11.59,23.97 11.59,25.88 v13.02,27.3
  Bottom 0.3: v13.02,27.3 13.02,28.1 12.79,28.32 R23.1
  Bottom 0.406: R20.2 6.64,28.32 R23.1
N$34  (via drill 0.3)
  Top 0.3: IC3.42 16.13,21.53 v15.72,21.11
  Bottom 0.3: v15.72,21.11 15.4,20.95 14.92,20.48 14.83,20.57 R19.2
N$35
  Bottom 0.406: C60.1 9.71,26.92 R23.2
N$36
  Bottom 0.406: C59.1 11.11,31.53 11.11,32.93 R22.2
N$37
  Bottom 0.406: C60.2 R24.2 6.15,24.82 X3.RIGHT
N$38
  Bottom 0.406: C59.2 10.16,34.42 X3.LEFT 8.62,33.43 R25.2
N$39
  Bottom 0.3: C61.1 14.61,23.1 R19.1
N$40
  Bottom 0.406: C62.1 3.43,26.42 R20.1
N$41
  Bottom 0.406: R21.1 C63.1
N$42  (via drill 0.4)
  Top 0.3: C64.1 18.16,8.26 IC3.1 12.45,17.08 v12.38,17.14
  Bottom 0.3: v12.38,17.14 12.38,19.75 R30.1
  Bottom 0.406: R30.1 12.29,20.82 C71.1
N$43
  Top 0.3: IC3.2 18.67,9.27 19.05,8.89 19.05,5.33 C65.1
N$44  (via drill 0.4)
  Top 0.406: C64.2 11.75,8.1 10.95,7.3 v10.48,7.3
  Bottom 0.406: 9.62,7.3 R27.1 X4.LEFT | 9.62,7.3 9.62,6.89 C66.1 | v10.48,7.3 9.62,7.3
N$45  (via drill 0.4)
  Top 0.406: C65.2 v10,4.6
  Bottom 0.406: C66.2 R28.2 | X4.GND 2.19,5.49 C66.2 | v10,4.6 9.53,5.08 8.57,5.08 C66.2
N$46  (via drill 0.4)
  Top 0.406: C67.2 14.67,5.56 v12.54,5.56
  Bottom 0.406: R29.2 7.27,3.11 R28.1 10.1,3.11 v12.54,5.56
N$47  (via drill 0.4)
  Top 0.406: v12.54,7.3 12.79,7.05 C67.1 C68.1
  Bottom 0.406: R26.1 11.27,8.57 R27.2 11.91,8.57 12.54,7.94 v12.54,7.3
N$48  (via drill 0.4)
  Top 0.3: IC3.48 11.97,18.48 11.27,17.78 11.27,14.92 v10.95,14.61
  Bottom 0.3: v10.95,14.61 8.96,14.61 C72.1
  Bottom 0.406: R31.1 C72.1
N$49
  Bottom 0.406: C69.2 9.84,22.44 X5.LEFT
N$50
  Bottom 0.406: C70.2 5.08,13.1 X5.RIGHT
N$51
  Bottom 0.406: C69.1 10.82,19.78 R30.2
N$52
  Bottom 0.406: C70.1 R31.2
N$53
  Top 0.3: IC3.23 25.86,23.56 26.04,23.73 26.04,24.53 24.77,25.8 24.77,27.62 25.24,28.1 28.89,28.1 30.24,29.45 30.24,32.23 29.92,32.54 IC8.16
N$54
  Top 0.3: R32.2 86.68,70.17 84.25,72.59 82.07,72.55 X6.10
N$55
  Top 0.3: R33.2 87.79,69.85 84.14,73.5 83.19,73.5 81.44,75.25 73.39,75.25 X6.11
N$56
  Top 0.7: X6.SHD@1 X6.SHD@0 68.26,66.26 L6.2
N$57  (via drill 0.3)
  Top 0.3: IC8.18 v28.73,30 | v25.4,16.67 25.4,18.22 IC3.13
  Bottom 0.3: v28.73,30 28.73,17.3 28.1,16.67 v25.4,16.67
N$58  (via drill 0.4)
  Top 0.3: IC8.3 31.27,30 31.27,25.4 30.96,25.08 v27.3,25.08 | IC3.3 19.18,17.81 18.89,18.1 18.89,19.21 19.53,19.84 v19.53,22.7
  Bottom 0.3: v19.53,22.7 20.48,22.7 21.59,23.81 21.59,24.45 22.07,24.92 22.86,24.92 23.97,26.04 26.35,26.04 v27.3,25.08
N$59
  Top 0.3: IC3.29 21.72,27.27 22.23,27.78 22.23,37.31 22.54,37.62 IC8.12
N$60
  Top 0.3: IC3.28 22.23,26.99 22.7,27.46 22.7,34.61 23.18,35.08 IC8.14
PB0
  Top 0.3: IC1.19 26.05,51.77 X17.2
PB1  (via drill 0.3)
  Top 0.3: IC1.20 28.09,51.27 X17.1 | IC8.6 33.26,33.81 31.51,35.56 31.51,38.42 27.94,41.99 v27.94,43.5
  Bottom 0.3: v27.94,43.5 27.94,46.99 26.91,48.02 24.84,48.02 X17.1
PB2  (via drill 0.3)
  Top 0.3: IC1.21 28.7,50.77 26.51,48.58 26.51,47.15 X17.4 | IC8.8 33.1,36.35 32.31,37.15 32.31,39.05 v28.97,42.39
  Bottom 0.3: v28.97,42.39 25.4,42.39 24.77,43.02 X17.4
PB3
  Top 0.3: IC1.22 29,50.27 27.15,48.42 27.15,45.4 25.4,43.66 23.97,43.66 | 23.97,43.66 X17.5 | IC3.30 21.21,28.11 21.75,28.65 21.75,41.43 23.97,43.66
PB4  (via drill 0.3)
  Top 0.3: IC1.23 29.84,49.77 v29.84,46.2
  Bottom 0.3: v29.84,46.2 29.84,40.32 31.43,40.32 31.43,33.18 35.08,33.18 35.08,29.69 34.13,29.69 34.13,18.89 30.16,14.92 29.05,14.92 25.24,11.11 25.24,8.57 X7.2
PB5  (via drill 0.3)
  Top 0.3: IC1.24 30.8,49.27 v30.8,46.99
  Bottom 0.3: v30.8,46.99 30.8,40.8 31.91,40.8 31.91,33.66 35.72,33.66 35.72,29.21 34.61,29.21 34.61,18.41 30.32,14.13 29.21,14.13 27.15,12.06 X7.1
PB6  (via drill 0.3)
  Top 0.3: IC1.25 31.75,48.77 v31.75,46.2
  Bottom 0.3: v31.75,46.2 31.75,41.27 32.38,41.27 32.38,34.13 36.35,34.13 36.35,28.73 35.24,28.73 35.24,18.26 30.48,13.49 30,13.49 29.69,13.18 X7.4
PB7  (via drill 0.3)
  Top 0.3: IC1.26 34.19,46.89 v32.7,45.4
  Bottom 0.3: v32.7,45.4 32.7,41.75 32.86,41.75 32.86,34.61 36.83,34.61 36.83,28.26 35.72,28.26 35.72,17.94 31.27,13.49 31.27,8.26 X7.5
PD0  (via drill 0.3)
  Top 0.3: IC1.43 44.38,47.85 43.97,48.26 43.97,51.59 46.2,53.82 46.2,55.88 v48.26,57.94
  Bottom 0.3: v48.26,57.94 51.28,57.94 53.02,59.69 X8.1
PD1  (via drill 0.3)
  Top 0.3: IC1.44 44.88,48.14 44.45,48.58 44.45,51.28 46.67,53.5 46.67,55.24 v48.26,56.83
  Bottom 0.3: v48.26,56.83 50.96,56.83 55.56,61.44 X8.2
PD2  (via drill 0.3)
  Top 0.3: IC1.45 45.38,48.44 44.93,48.9 44.93,50.8 46.04,51.91 v48.42,51.91 | v74.93,44.61 74.93,41.27 75.45,40.75 IC2.65
  Bottom 0.3: v48.42,51.91 49.05,51.91 49.37,51.59 61.12,51.59 64.45,54.93 69.22,54.93 70.33,53.82 70.33,46.04 70.8,45.56 73.98,45.56 v74.93,44.61
PD3  (via drill 0.3)
  Top 0.3: IC3.8 21.72,15.84 21.27,15.4 20.16,15.4 19.68,14.92 19.68,12.06 20,11.75 25.56,11.75 26.19,12.38 26.19,15.88 26.99,16.67 34.92,16.67 37.78,19.53 v37.78,23.81 | IC1.46 45.88,49.21 v45.72,49.37
  Bottom 0.3: v45.72,49.37 45.72,42.86 46.35,42.23 46.35,37.62 45.56,36.83 39.53,36.83 38.73,36.04 38.73,24.77 v37.78,23.81
PD4  (via drill 0.3)
  Top 0.3: IC1.47 46.38,49.66 45.88,50.16 45.88,50.64 46.35,51.12 v48.42,51.12 | IC2.66 75.95,42.16 v75.72,42.39
  Bottom 0.3: v48.42,51.12 61.44,51.12 64.77,54.45 68.9,54.45 69.85,53.5 69.85,45.72 70.48,45.09 73.03,45.09 v75.72,42.39
PD5  (via drill 0.3, 0.4)
  Top 0.3: IC8.17 v28.73,31.27 | v32.07,31.27 32.54,31.91 v39.85,31.91 | IC1.48 46.88,50.11 v46.83,50.16
  Bottom 0.3: v28.73,31.27 v32.07,31.27 | v46.83,50.16 46.83,37.31 45.88,36.35 39.85,36.35 39.21,35.72 39.21,32.54 v39.85,31.91
PD6  (via drill 0.3)
  Top 0.3: IC1.49 47.38,48.34 47.62,48.58 v47.62,48.9 | v40.8,31.27 IC8.4
  Bottom 0.3: v47.62,48.9 47.62,48.58 47.31,48.26 47.31,36.99 46.2,35.88 40.32,35.88 40.01,35.56 40.01,32.86 40.8,32.07 v40.8,31.27
PD7  (via drill 0.3)
  Top 0.3: IC1.50 49.15,46.89 v49.21,46.83 | v40.8,28.73 IC8.2
  Bottom 0.3: v49.21,46.83 49.21,45.56 47.78,44.13 47.78,36.67 46.51,35.4 42.07,35.4 41.59,34.92 41.59,29.53 v40.8,28.73
PE0
  Top 0.3: IC1.2 32.92,60.27 29.69,63.5 16.83,63.5 16.67,63.66 16.67,64.14 15.4,65.41 8.89,65.41 X9.4
PE1
  Top 0.3: IC1.3 32.62,59.77 29.37,63.02 16.51,63.02 16.19,63.34 16.19,63.82 15.08,64.93 10.95,64.93 X9.3
PE2
  Top 0.3: IC1.4 32.33,59.27 29.05,62.55 16.03,62.55 15.72,62.87 15.72,63.5 14.76,64.45 13.02,64.45 X9.2
PE3
  Top 0.3: IC1.5 32.04,58.77 28.73,62.07 15.08,62.07 X9.1
PE4
  Top 0.3: IC1.6 31.74,58.27 28.57,61.44 15.08,61.44 X9.6
PE5
  Top 0.3: IC1.7 31.45,57.77 28.26,60.96 16.03,60.96 15.72,60.64 15.72,60.01 14.76,59.05 13.02,59.05 X9.7
PE6
  Top 0.3: IC1.8 31.16,57.27 27.94,60.48 16.51,60.48 16.19,60.17 16.19,59.69 15.08,58.58 10.95,58.58 X9.8
PE7
  Top 0.3: IC1.9 30.86,56.77 27.62,60.01 16.99,60.01 16.67,59.69 16.67,59.37 15.4,58.1 8.89,58.1 X9.9
PG3  (via drill 0.3)
  Top 0.3: IC1.28 36.88,45.77 36.2,45.09 35.4,45.09 34.29,43.97 v34.29,40.48
  Bottom 0.3: v34.29,40.48 34.29,35.24 37.31,35.24 37.31,27.78 36.2,27.78 36.2,11.91 34.13,9.84 34.13,8.41 X18.2
PG4  (via drill 0.3)
  Top 0.3: IC1.29 37.38,45.32 36.51,44.45 35.72,44.45 35.24,43.97 v35.24,40.16
  Bottom 0.3: v35.24,40.16 35.24,35.72 37.78,35.72 37.78,27.3 36.67,27.3 36.67,10.16 X18.1
PG5  (via drill 0.3)
  Top 0.3: IC1.1 35.43,60.77 35.72,60.48 35.72,59.53 36.99,58.26 36.99,55.56 v41.27,51.28 | v38.58,37.94 38.58,35.88 40.64,33.81 40.64,33.02 41.91,31.75 41.91,17.78 40.01,15.88 40.01,12.22 38.42,12.22 X18.4
  Bottom 0.3: v41.27,51.28 41.27,48.74 39.05,46.51 35.4,46.51 34.29,45.4 34.29,42.23 v38.58,37.94
PH0
  Top 0.3: IC1.12 31.57,55.27 31.11,55.72 16.83,55.72 16.67,55.88 16.67,56.36 15.4,57.63 8.89,57.63 X10.4
PH1
  Top 0.3: IC1.13 31.27,54.77 30.8,55.24 16.51,55.24 16.19,55.56 16.19,56.04 15.08,57.15 10.95,57.15 X10.3
PH2
  Top 0.3: IC1.14 30.98,54.27 30.48,54.77 16.03,54.77 15.72,55.09 15.72,55.72 14.76,56.67 13.02,56.67 X10.2
PH3
  Top 0.3: IC1.15 30.69,53.77 30.16,54.29 15.08,54.29 X10.1
PH4
  Top 0.3: IC1.16 30.39,53.27 30,53.66 15.08,53.66 X10.6
PH5
  Top 0.3: IC1.17 30.1,52.77 29.69,53.18 16.03,53.18 15.72,52.86 15.72,52.23 14.76,51.28 13.02,51.28 X10.7
PH6
  Top 0.3: IC1.18 29.8,52.27 29.37,52.7 16.51,52.7 16.19,52.39 16.19,51.91 15.08,50.8 11.11,50.8 X10.8
PH7  (via drill 0.3)
  Top 0.3: X10.9 8.89,50.32 15.4,50.32 16.67,51.59 16.67,52.07 16.83,52.23 22.38,52.23 v23.34,51.28 | 36.35,51.12 v36.2,51.28 36.38,51.09 IC1.27
  Bottom 0.3: v23.34,51.28 v36.2,51.28
PJ0  (via drill 0.3)
  Top 0.3: IC1.63 50.8,54.77 v51.28,54.29
  Bottom 0.3: v51.28,54.29 59.69,54.29 61.75,56.36 X11.4
PJ1  (via drill 0.3)
  Top 0.3: IC1.64 51.25,55.27 v51.44,55.09
  Bottom 0.3: v51.44,55.09 51.75,54.77 59.37,54.77 61.28,56.67 61.28,70.64 X11.3
PJ2  (via drill 0.3)
  Top 0.3: IC1.65 51.86,55.77 v52.07,55.56
  Bottom 0.3: v52.07,55.56 52.39,55.24 59.05,55.24 60.8,56.99 60.8,70.33 60.01,71.12 58.26,71.12 X11.2
PJ3  (via drill 0.3)
  Top 0.3: IC1.66 52.48,56.27 v52.7,56.04
  Bottom 0.3: v52.7,56.04 53.02,55.72 58.74,55.72 60.33,57.31 60.33,70.01 59.69,70.64 56.2,70.64 X11.1
PJ4  (via drill 0.3)
  Top 0.3: IC1.67 53.09,56.77 v53.34,56.52
  Bottom 0.3: v53.34,56.52 53.66,56.2 58.42,56.2 59.85,57.63 59.85,69.69 59.37,70.17 54.45,70.17 52.55,72.07 52.55,73.66 X11.6
PJ5  (via drill 0.3)
  Top 0.3: IC1.68 53.7,57.27 v53.98,56.99
  Bottom 0.3: v53.98,56.99 54.29,56.67 58.1,56.67 59.37,57.94 59.37,69.37 59.05,69.69 54.13,69.69 52.07,71.75 52.07,75.25 53.66,76.83 55.09,76.83 X11.7
PJ6  (via drill 0.3)
  Top 0.3: IC1.69 54.31,57.77 v54.61,57.47
  Bottom 0.3: v54.61,57.47 54.93,57.15 57.78,57.15 58.9,58.26 58.9,69.06 58.74,69.22 53.82,69.22 51.59,71.44 51.59,75.56 53.34,77.31 57.15,77.31 X11.8
PJ7
  Top 0.3: IC1.79 46.41,66.09 47.31,66.99 51.28,66.99 52.23,67.94 52.23,75.72 53.5,76.99 60.01,76.99 X11.9
PL0
  Top 0.3: IC1.35 40.38,43.44 41.59,42.23 46.2,42.23 46.83,41.59 46.83,40.64 46.04,39.85 46.04,31.59 45.88,31.43 45.24,31.43 44.13,30.32 44.13,23.81 X12.4
PL1
  Top 0.3: IC1.36 40.88,43.73 41.91,42.7 46.51,42.7 47.31,41.91 47.31,40.32 46.51,39.53 46.51,31.27 46.2,30.96 45.56,30.96 44.61,30 44.61,25.88 X12.3
PL2
  Top 0.3: IC1.37 41.38,44.02 42.23,43.18 46.83,43.18 47.78,42.23 47.78,40.01 46.99,39.21 46.99,30.8 46.67,30.48 45.88,30.48 45.09,29.69 45.09,27.94 X12.2
PL3
  Top 0.3: IC1.38 41.88,44.32 42.55,43.66 47.15,43.66 48.26,42.55 48.26,39.69 47.47,38.89 47.47,30 X12.1
PL4
  Top 0.3: IC1.39 42.38,44.61 42.86,44.13 47.47,44.13 48.74,42.86 48.74,39.37 48.1,38.73 48.1,30 X12.6
PL5
  Top 0.3: IC1.40 42.88,45.22 43.5,44.61 47.78,44.61 49.21,43.18 49.21,39.05 48.58,38.42 48.58,30.8 48.9,30.48 49.69,30.48 50.48,29.69 50.48,27.94 X12.7
PL6
  Top 0.3: IC1.41 43.38,45.52 43.81,45.09 48.1,45.09 49.69,43.5 49.69,38.73 49.05,38.1 49.05,31.27 49.37,30.96 50.01,30.96 50.96,30 50.96,25.88 X12.8
PL7
  Top 0.3: IC1.42 43.88,45.97 44.29,45.56 48.42,45.56 50.16,43.81 50.16,38.42 49.53,37.78 49.53,31.59 49.69,31.43 50.32,31.43 51.44,30.32 51.44,23.81 X12.9
RXIN  (via drill 0.3)
  Top 0.3: IC2.6 77.95,55.87 v77.63,56.2
  Bottom 0.3: X6.6 76.76,59.93 R5.1 76.76,56.43 76.99,56.2 v77.63,56.2
RXIP  (via drill 0.3)
  Top 0.3: IC2.5 78.45,55.85 v78.58,56.2
  Bottom 0.3: X6.3 79.06,60.8 78.18,59.93 R4.1 78.11,58.5 78.11,56.67 v78.58,56.2
SRAM  (via drill 0.3)
  Top 0.3: IC4.20 v68.74,14.61 | v54.29,5.4 IC6.11 | IC7.10 IC7.9 v67.79,8.57
  Bottom 0.3: v68.74,14.61 68.74,12.7 67.94,12.7 67.79,12.7 | 67.79,12.7 59.05,12.7 59.05,7.94 54.29,7.94 v54.29,5.4 | v67.79,8.57 67.79,12.7
TXON
  Top 0.3: X6.2 78.98,60.09 R7.2 78.98,57.71 78.58,57.31 76.68,57.31 76.52,57.15 76.45,57.05 IC2.9
TXOP
  Top 0.3: X6.1 81.6,60.8 80.41,59.61 R6.2 80.41,57.39 79.85,56.83 76.99,56.83 76.95,56.71 IC2.8
VCC  (via drill 0.3, 0.7)
  Top 0.3: IC1.10 35.47,56.27 v35.56,56.36 | IC1.61 48.37,53.77 v48.26,53.66 | IC1.80 45.91,61.15 v45.88,61.12 | IC1.31 38.38,48.55 v38.42,48.58 | C28.1 IC4.28 | C30.1 58.1,2.48 IC6.14 v58.1,5.4 | IC7.14 59.85,10.06 C31.1 v59.85,8.89 | C29.1 IC5.20
  Top 0.55: IC4.28 v70.96,4.45 | IC4.28 77.47,4.45 79.38,2.54 86.04,2.54 87.31,3.81 87.31,12.06 88.58,13.34 88.58,22.86 81.44,30 v81.44,31.59 | v78.74,31.59 77.15,31.59 76.14,32.61 C29.1
  Top 0.7: X17.3 17.46,47.94 15.48,45.96 C1.1 10.24,46.04 BR1.2 6.35,46.04 v7.78,44.61 | X9.5 2.7,63.02 1.75,62.07 1.75,57.47 X10.5 | X7.3 29.05,2.22 34.29,2.38 X18.3 | v43.81,32.54 44.61,32.54 44.83,32.77 R2.1 | X11.5 64.29,68.9 63.18,67.79 v54.93,67.79 | v40.48,25.72 33.81,25.72 33.81,28.42 v33.18,29.05
  Bottom 0.3: v35.56,56.36 C33.1 36.45,55.4 | v48.26,53.66 C35.1 | C36.1 v45.88,61.12 42.86,61.12 40.32,63.66 40.32,66.67 36.2,70.8 31.75,70.8 30.8,71.75 30.8,75.88 29.84,76.83 23.02,76.83 X15.7 | v38.42,48.58 C34.1 | 59.85,6.51 v59.85,8.89
  Bottom 0.55: v81.44,31.59 v78.74,31.59
  Bottom 0.7: C34.1 37.69,49.47 37.4,49.59 37.4,55.31 | 36.45,55.4 37.31,55.4 37.4,55.31 | C33.1 36.35,56.26 36.35,54.29 35.4,53.34 22.86,53.34 19.68,50.16 X17.3 17.3,45.56 17.3,42.86 19.37,42.86 20.48,41.75 23.34,41.75 24.13,40.96 26.67,40.96 30.32,37.31 30.32,33.02 31.11,32.23 33.02,32.23 33.66,31.59 33.66,31.11 33.18,30.64 v33.18,29.05 | v7.78,44.61 1.91,50.48 1.91,53.18 X10.5 | 37.4,55.31 40.39,55.31 42.07,56.99 | 42.07,56.99 42.07,59.56 42.13,59.62 42.48,60.07 C36.1 47.21,60.07 51.91,64.77 53.5,64.77 54.93,66.2 v54.93,67.79 | 42.07,56.99 46.35,56.99 47.47,55.88 47.47,53.75 C35.1 | v70.96,4.45 59.85,4.45 59.85,6.51 58.1,6.51 v58.1,5.4 58.1,3.49 56.83,2.22 50.64,2.22 48.74,4.13 45.09,4.13 | X18.3 37.94,2.06 43.02,2.06 45.09,4.13 | 45.09,4.13 45.09,17.46 X12.5 44.93,20.48 44.93,22.38 43.81,23.5 43.81,25.72 | 43.81,25.72 v43.81,32.54 | 43.81,25.72 v40.48,25.72
VCC1A8  (via drill 0.3, 0.7)
  Top 0.3: IC2.7 77.47,54.23 v77.47,52.23 | IC2.17 72.45,52.29 v72.39,52.23
  Top 0.7: L4.2 91.19,60.81 C14.1 90.73,61.04 90.65,61.12 v88.9,61.12
  Bottom 0.3: v77.47,52.23 C15.1 | C74.1 v72.39,52.23 73.18,53.02 76.68,53.02 v77.47,52.23 | v77.47,52.23 77.95,52.23 79.22,53.5 82.23,53.5 87.31,58.58 87.31,59.53 v88.9,61.12
VCC1V8  (via drill 0.3, 0.7)
  Top 0.3: IC2.11 75.45,52.28 v75.41,52.23 75.41,46.04 | IC2.92 80.9,48.35 v80.64,48.1 | IC2.94 80.95,49.35 v80.8,49.21 80.64,49.05 v80.64,48.1 | IC2.58 71.95,40.12 v71.91,40.16 71.91,46.04 | IC2.72 78.95,40.06 v78.9,40.16 78.9,46.04 | IC2.36 68.19,47.38 v68.26,47.31 69.53,46.04 71.91,46.04 | v80.64,48.1 79.38,48.1 78.9,47.62 78.9,46.04 | 75.41,46.04 71.91,46.04 | 78.9,46.04 75.41,46.04
  Top 0.7: BR8.2 BR7.2 92.71,68.66 C7.1 C11.1 92.63,65.58 C12.1 C13.1 92.55,64.2 L4.1 93.67,63.01 93.82,62.87 93.82,60.01 v92.71,58.9
  Bottom 0.3: v75.41,52.23 C46.1 | v80.64,48.1 C50.1 | v80.8,49.21 81.69,49.21 C51.1 | v71.91,40.16 C48.1 | v78.9,40.16 C49.1 | v68.26,47.31 C47.1
  Bottom 0.7: v92.71,58.9 90.65,58.9 83.82,52.07 82.71,52.07 81.76,51.12 81.76,49.47 C51.1
VCC3A3  (via drill 0.3)
  Top 0.3: IC2.2 79.95,52.33 v79.85,52.23
  Top 0.7: L2.2 96.27,60.97 C10.1 96.04,59.85 v95.25,59.05
  Bottom 0.3: v79.85,52.23 79.85,51.12 | 79.85,51.12 C75.1 | v95.25,59.05 94.61,59.05 93.34,60.33 90.49,60.33 83.34,53.18 82.71,53.18 82.39,52.86 81.44,52.86 80.64,52.07 80.64,51.91 79.85,51.12
VCC3V3  (via drill 0.3)
  Top 0.3: X6.9 82.03,76.68 72.39,76.68 70.83,75.11 X6.12 66.2,69.08 66.2,59.37 66.67,58.9 66.67,52.48 IC2.26 v68.25,52.38 | IC2.14 73.95,52.25 v73.98,52.23 73.98,51.12 70.01,51.12 70.01,52.38 v68.25,52.38 | IC2.83 80.69,43.85 v80.64,43.81 | IC2.63 v74.45,40.16 | IC2.46 v68.26,42.38 v68.26,42.39 | v68.25,52.38 v68.26,52.39 | BR3.2 97.79,63.34 97.63,63.18
  Top 0.7: BR3.2 97.79,67.7 C3.1 C8.1 97.71,64.63 C9.1 97.63,64.36 97.63,63.18 | L2.1 97.63,63.18 | 97.63,63.18 98.9,63.18 99.22,62.87 99.22,59.85 98.74,59.37 v97.47,59.37
  Bottom 0.3: v73.98,52.23 C41.1 | C45.1 v80.64,43.81 79.53,43.81 77.47,41.75 74.93,41.75 74.45,41.27 | C44.1 v74.45,40.16 74.45,41.27 | v68.26,42.39 C43.1 | C42.1 v68.26,52.39 68.26,50.48 69.37,49.37 69.37,43.5 v68.26,42.39 | 74.45,41.27 73.98,41.75 68.9,41.75 v68.26,42.39
  Bottom 0.7: v97.47,59.37 88.9,50.8 88.9,46.51 87.31,44.93 81.76,44.93 81.76,43.91 C45.1
W5300  (via drill 0.3)
  Top 0.3: IC7.6 67.79,1.59 v70.48,1.59 | v76.68,36.67 73.95,36.67 IC2.62
  Bottom 0.3: v70.48,1.59 72.07,3.17 83.66,3.17 85.25,4.76 85.25,10.95 87.63,13.34 87.63,20.16 76.68,31.11 v76.68,36.67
